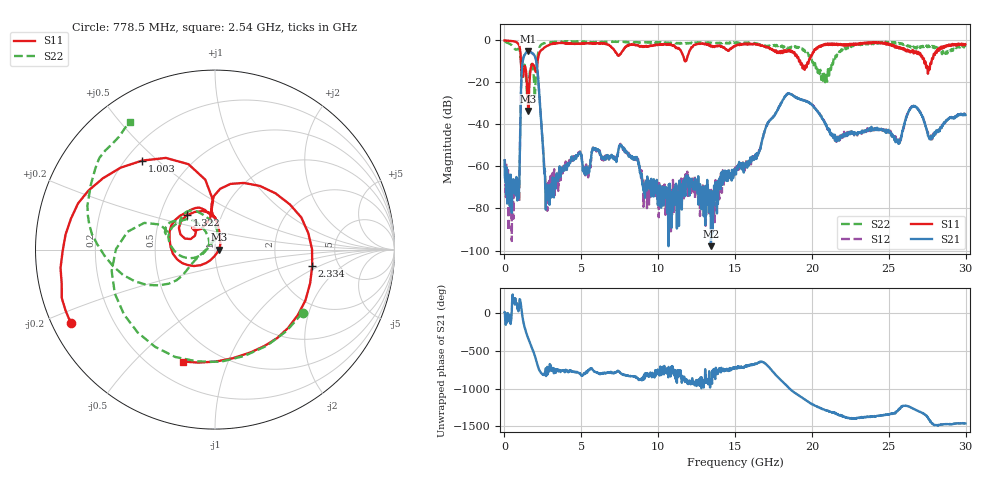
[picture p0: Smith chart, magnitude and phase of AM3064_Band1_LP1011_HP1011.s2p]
# Hz S DB R 50.0
!freq dBS11 angS11 dBS21 angS21 dBS12 angS12 dBS22 angS22
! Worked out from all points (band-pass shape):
!   1600 points, 10 MHz to 29.98 GHz, reference 50 ohm
!   highest |S21| = -5.13 dB at 1.528 GHz (marker M1); lowest = -97.9 dB at 13.43 GHz (marker M2)
!   |S21| within 3 dB of the highest: 1.24 GHz to 2.008 GHz (767.9 MHz wide, 47.3 % of centre)
!   lowest |S11| = -33.6 dB at 1.547 GHz (marker M3), VSWR 1.04, Z = 52.1 + j0.043 ohm
!   |S11| at or under -10 dB: 1.071 GHz to 2.155 GHz (1.084 GHz wide, 67.2 % of centre); 19.24 GHz to 19.79 GHz (550.7 MHz wide, 2.82 % of centre); 27.3 GHz to 27.78 GHz (478.9 MHz wide, 1.74 % of centre)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
!   |S22| runs from -28.8 to -0.3 dB; largest |S21 - S12| = 0.0068
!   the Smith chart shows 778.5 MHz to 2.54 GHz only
!   S11 on the Smith chart (normalised r, x): 778.5 MHz: 0.05, -0.24; 1.003 GHz: 0.27, +0.45; 1.322 GHz: 0.68, +0.28; 2.334 GHz: 3.20, -0.82; 2.54 GHz: 0.33, -0.70
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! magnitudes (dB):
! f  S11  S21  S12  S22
! 10 MHz  0.0  -57.1  -56.5  -0.3
! 778.5 MHz  -0.9  -65.0  -72.0  -4.4
! 1.003 GHz  -3.9  -50.8  -51.3  -5.2
! 1.322 GHz  -12.1  -6.8  -6.7  -11.9
! 1.528 GHz  -29.5  -5.1  -5.1  -24.5
! 1.547 GHz  -33.6  -5.2  -5.1  -22.3
! 2.034 GHz  -14.9  -8.7  -8.7  -17.8
! 2.334 GHz  -5.2  -32.9  -32.8  -2.5
! 2.54 GHz  -3.8  -54.3  -54.1  -1.4
! 2.84 GHz  -2.4  -72.0  -73.9  -0.9
! 5.015 GHz  -1.4  -54.6  -55.8  -0.8
! 7.639 GHz  -5.4  -50.4  -50.6  -0.7
! 10 GHz  -2.1  -69.2  -72.6  -1.0
! 13.43 GHz  -2.7  -97.9  -77.7  -1.4
! 15 GHz  -2.6  -62.2  -60.6  -1.4
! 18.34 GHz  -5.5  -25.9  -25.8  -3.4
! 19.99 GHz  -7.3  -30.5  -30.5  -9.3
! 21.57 GHz  -2.1  -45.8  -45.9  -7.4
! 25 GHz  -1.5  -43.3  -42.8  -1.0
! 26.66 GHz  -5.3  -31.4  -31.2  -3.6
! 27.56 GHz  -15.1  -45.4  -44.9  -2.5
! 29.98 GHz  -1.8  -35.5  -35.5  -3.0
